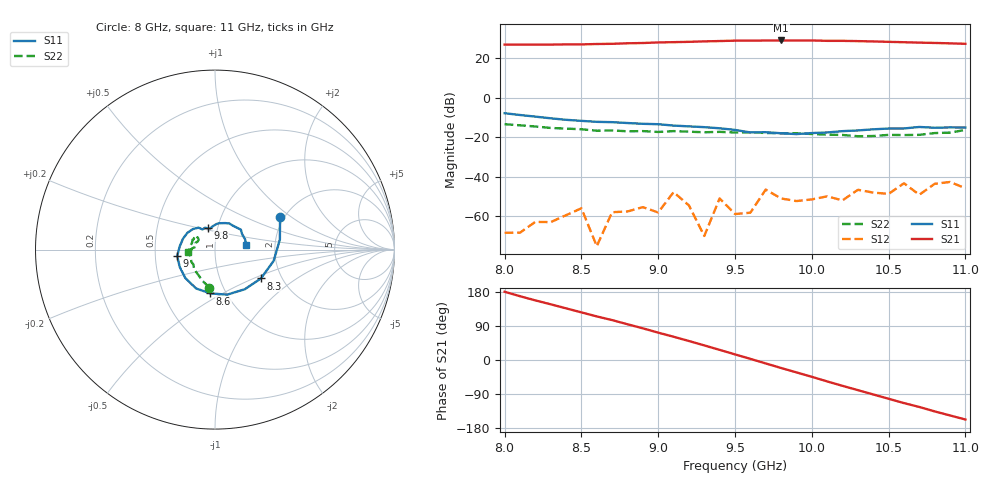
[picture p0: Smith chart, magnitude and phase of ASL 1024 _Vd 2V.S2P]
! AWR Design Environment (7688) Tue Apr 11 16:29:48 2017
! Document = 'ASL 1024  Vd 2V'
! nPorts: 2, nXvals: 31
# HZ S DB R 50
!Freq DBS11 AngS11 DBS21 AngS21 DBS12 AngS12 DBS22 AngS22
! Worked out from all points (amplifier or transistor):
!   31 points, 8 GHz to 11 GHz, reference 50 ohm
!   highest |S21| = 29.1 dB at 9.8 GHz (marker M1)
!   |S21| within 3 dB of that: start of sweep to end of sweep
!   unconditionally stable (mu >= 1): start of sweep to end of sweep
!   at 8.5 GHz: K = 12.77, MAG = 27.5 dB, |S12| = -56.1 dB
!   at 9.5 GHz: K = 15.17, MAG = 29.2 dB, |S12| = -59.0 dB
!   at 11 GHz: K = 4.07, MAG = 27.6 dB, |S12| = -45.9 dB
!   lowest NFmin = 0.00 dB at 8 GHz
!   S11 on the Smith chart (normalised r, x): 8 GHz: 1.90, +0.83; 8.3 GHz: 1.57, -0.55; 8.6 GHz: 0.84, -0.44; 9 GHz: 0.65, -0.05; 9.8 GHz: 0.90, +0.22; 11 GHz: 1.42, +0.07
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8e9  -7.83 26.8  27.00 180.0  -68.50 -174.0  -13.40 -99.0
8.1e9  -8.73 9.0  27.00 168.3  -68.45 114.6  -13.97 -104.0
8.3e9  -10.40 -32.2  27.00 147.0  -63.10 -97.3  -15.30 -121.0
8.5e9  -11.70 -74.9  27.10 125.7  -56.07 87.9  -15.96 -137.3
8.6e9  -12.20 -96.1  27.30 115.0  -75.30 38.5  -16.70 -145.0
8.8e9  -12.80 -136.3  27.67 94.3  -57.68 84.2  -17.00 -162.3
9e9  -13.40 -170.3  28.10 72.1  -58.18 51.1  -17.34 -179.3
9.1e9  -14.10 174.7  28.23 61.4  -47.89 -4.8  -16.90 179.3
9.3e9  -14.90 148.7  28.63 38.5  -70.14 -3.0  -17.50 163.0
9.4e9  -15.47 137.4  28.80 26.8  -51.06 -110.4  -17.28 156.3
9.5e9  -16.30 127.0  29.00 14.8  -59.00 -82.4  -17.60 154.0
9.6e9  -17.58 121.7  29.00 3.0  -58.32 -163.9  -17.50 151.7
9.7e9  -17.46 114.7  29.07 -9.1  -46.59 -110.3  -17.87 145.3
9.8e9  -18.00 109.0  29.10 -21.1  -51.10 -107.0  -18.00 147.0
1e10  -17.90 98.0  29.10 -44.4  -51.56 -110.1  -18.37 145.3
1.02e10  -16.92 86.7  28.90 -68.2  -52.06 -134.1  -18.87 146.0
1.03e10  -16.56 81.5  28.77 -79.6  -46.69 -174.0  -19.50 149.2
1.04e10  -16.00 68.8  28.60 -90.9  -48.10 -140.0  -19.40 156.0
1.05e10  -15.60 61.2  28.40 -102.3  -48.77 -164.2  -18.83 160.8
1.07e10  -14.80 37.6  28.00 -124.0  -49.20 -142.0  -18.80 174.0
1.08e10  -15.20 29.2  27.83 -135.7  -43.67 169.0  -17.90 176.7
1.1e10  -15.10 7.9  27.40 -157.0  -45.90 172.0  -16.30 -175.0
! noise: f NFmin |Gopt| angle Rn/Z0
8e+09  0  1  0  2e-20
8.3e+09  0  1  0  2e-20
8.6e+09  0  1  0  2e-20
9e+09  0  1  0  2e-20
9.3e+09  0  1  0  2e-20
9.6e+09  0  1  0  2e-20
1e+10  0  1  0  2e-20
1.03e+10  0  1  0  2e-20
1.06e+10  0  1  0  2e-20
1.1e+10  0  1  0  2e-20
